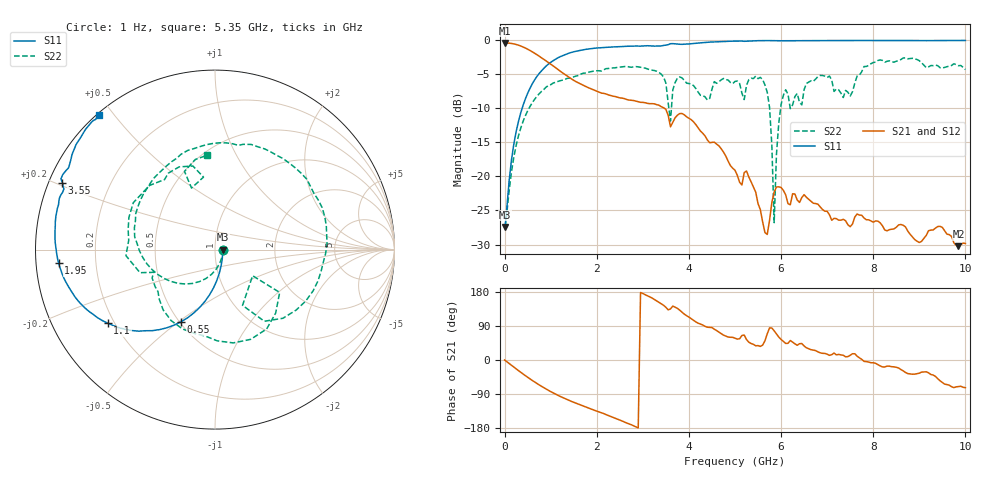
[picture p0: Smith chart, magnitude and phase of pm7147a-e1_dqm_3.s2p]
# GHz S DB R 50
! S-Parameters data
! Freq  dbS11  angS11  dbS21  angS21  dbS12  angS12  dbS22  angS22
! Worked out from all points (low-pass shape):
!   279 points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, 1 Hz to 10 GHz, reference 50 ohm
!   highest |S21| = -0.38 dB at 31.62 kHz (marker M1); lowest = -30.2 dB at 9.85 GHz (marker M2)
!   |S21| within 3 dB of the highest: start of sweep to 974.3 MHz
!   lowest |S11| = -27.4 dB at 31.62 kHz (marker M3), VSWR 1.09, Z = 54.4 - j0.00239 ohm
!   |S11| at or under -10 dB: start of sweep to 380.3 MHz
!   |S22| runs from -27.4 to -2.6 dB; largest |S21 - S12| = 1.6e-12
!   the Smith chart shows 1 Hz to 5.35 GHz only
!   S11 on the Smith chart (normalised r, x): 1 Hz: 1.09, -0.00; 550 MHz: 0.51, -0.51; 1.1 GHz: 0.17, -0.30; 1.95 GHz: 0.07, -0.04; 3.55 GHz: 0.04, +0.21; 5.35 GHz: 0.01, +0.46
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1e-09  -27.43 -0.0  -0.38 -0.0  -0.38 -0.0  -27.43 -0.0
3.16228e-05  -27.43 -0.0  -0.38 -0.0  -0.38 -0.0  -27.43 -0.0
0.55  -7.05 -115.2  -1.49 -49.8  -1.49 -49.8  -9.73 -150.5
1.1  -2.80 -145.5  -4.00 -89.7  -4.00 -89.7  -6.17 151.0
1.7  -1.40 -168.0  -6.57 -121.2  -6.57 -121.2  -4.84 105.4
1.95  -1.16 -175.1  -7.35 -132.7  -7.35 -132.7  -4.50 87.5
2.85  -0.84 165.7  -8.93 -176.6  -8.93 -176.6  -3.86 21.3
3.35  -0.85 158.2  -9.53 152.2  -9.53 152.2  -4.72 -29.6
3.55  -0.64 156.3  -11.03 132.3  -11.03 132.3  -9.21 -63.7
3.65  -0.49 153.8  -12.02 142.3  -12.02 142.3  -7.28 -33.5
3.9  -0.57 150.3  -10.94 121.0  -10.94 121.0  -5.88 -88.6
4.55  -0.25 141.5  -14.96 81.4  -14.96 81.4  -6.07 -176.1
5.05  -0.11 134.6  -19.82 55.2  -19.82 55.2  -5.98 113.5
5.35  -0.09 130.9  -20.80 43.5  -20.80 43.5  -5.57 95.0
5.7  -0.04 126.4  -28.52 69.2  -28.52 69.2  -7.63 29.8
5.85  -0.07 124.6  -22.28 77.0  -22.28 77.0  -26.79 -121.1
5.9  -0.07 124.1  -21.55 68.7  -21.55 68.7  -16.71 157.9
6.05  -0.06 122.5  -22.05 49.1  -22.05 49.1  -8.08 110.0
6.7  -0.04 115.8  -23.94 26.2  -23.94 26.2  -6.02 76.3
8.35  -0.03 101.2  -27.81 -16.2  -27.81 -16.2  -3.01 27.1
9.85  -0.02 90.7  -30.24 -70.0  -30.24 -70.0  -3.73 -28.5
10  -0.02 89.7  -29.85 -73.0  -29.85 -73.0  -4.29 -34.6
